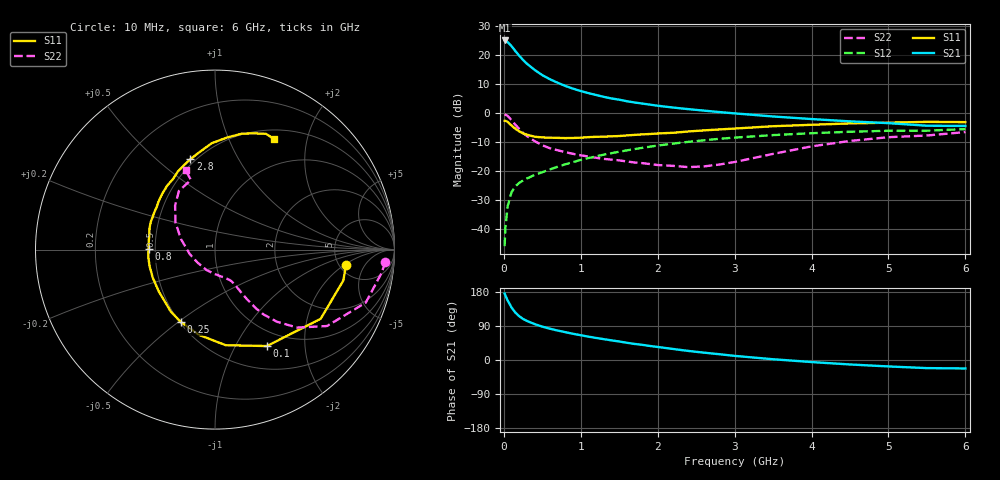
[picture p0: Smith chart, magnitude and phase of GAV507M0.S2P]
! Infineon Technologies  Discrete & RF Semiconductors
! BF775
! Si NPN RF Bipolar Junction Transistor in SOT23
! VCE = 0.5 V  IC = 7 mA
! Common Emitter S-Parameters:  May  1996
# GHz  S  MA  R  50
!  f  S11  S21  S12  S22
! GHz  MAG  ANG  MAG  ANG  MAG  ANG  MAG  ANG
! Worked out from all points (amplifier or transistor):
!   36 points, 10 MHz to 6 GHz, reference 50 ohm
!   highest |S21| = 25.0 dB at 10 MHz (marker M1)
!   |S21| within 3 dB of that: start of sweep to 130.4 MHz
!   unconditionally stable (mu >= 1): 477.1 MHz to end of sweep
!   at 250 MHz: K = 0.68, MSG = 20.8 dB, |S12| = -23.2 dB
!   at 1.4 GHz: K = 1.26, MAG = 6.4 dB, |S12| = -13.8 dB
!   at 6 GHz: K = 1.10, MAG = -1.4 dB, |S12| = -5.5 dB
!   S11 on the Smith chart (normalised r, x): 10 MHz: 5.69, -2.18; 100 MHz: 0.79, -1.35; 250 MHz: 0.51, -0.51; 800 MHz: 0.46, +0.00; 2.8 GHz: 0.47, +0.65; 6 GHz: 0.62, +1.49
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0.01  0.735 -6.9  17.78 175.3  0.0051 85.0  0.9519 -4.1
0.02  0.7355 -13.5  17.48 170.2  0.0106 81.3  0.9371 -8.0
0.05  0.7038 -33.2  16.67 157.0  0.0251 73.6  0.8903 -19.4
0.1  0.6102 -61.7  14.19 138.6  0.0433 62.2  0.7555 -34.3
0.15  0.5361 -83.6  11.65 125.1  0.0548 54.9  0.6311 -43.5
0.2  0.4829 -100.9  9.733 115.6  0.0626 51.6  0.5305 -49.3
0.25  0.4454 -115.5  8.202 108.2  0.069 50.2  0.4527 -53.1
0.3  0.4242 -125.5  7.074 103.1  0.0746 49.9  0.4016 -55.0
0.4  0.3911 -142.9  5.541 94.8  0.0858 50.5  0.3291 -57.2
0.5  0.3805 -155.7  4.491 88.0  0.0958 51.4  0.2786 -58.6
0.6  0.3762 -165.5  3.814 82.5  0.1071 52.7  0.2475 -59.6
0.8  0.3704 179.7  2.928 73.4  0.131 53.4  0.212 -61.4
0.9  0.3722 172.3  2.626 69.2  0.1434 53.4  0.1984 -62.5
1.1  0.3844 161.6  2.202 61.6  0.1676 53.1  0.1782 -67.0
1.3  0.3923 152.4  1.899 55.0  0.1923 51.8  0.1625 -71.9
1.6  0.4117 140.1  1.596 45.4  0.2279 49.1  0.1467 -81.6
2.2  0.457 120.9  1.243 29.1  0.2974 42.1  0.1231 -112.5
2.8  0.5219 105.2  1.04 15.3  0.3597 33.9  0.1297 -158.2
3.5  0.5929 91.8  0.873 2.0  0.417 23.8  0.1979 163.0
4.5  0.663 77.0  0.719 -11.8  0.4761 10.3  0.3309 132.2
5.5  0.705 66.2  0.605 -21.4  0.4966 -2.6  0.4105 109.1
6  0.6978 61.7  0.599 -22.3  0.529 -6.3  0.4704 110.2
